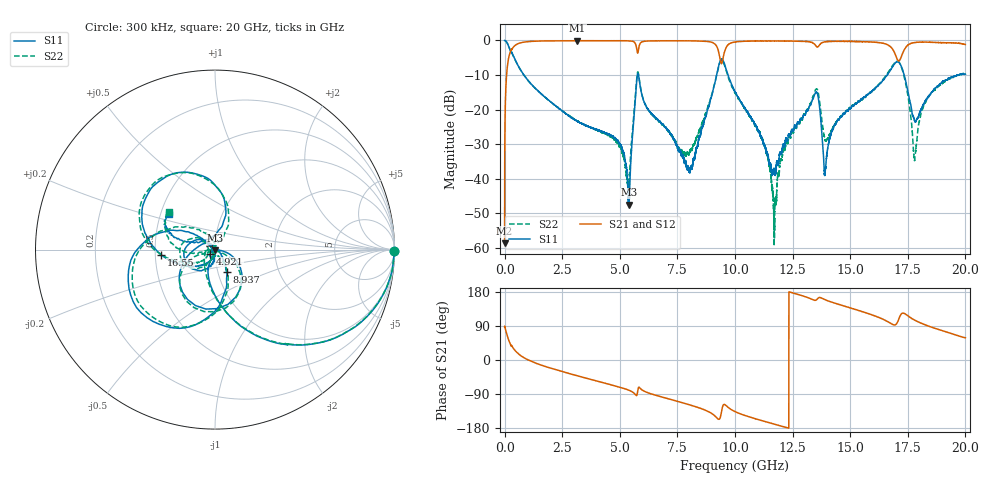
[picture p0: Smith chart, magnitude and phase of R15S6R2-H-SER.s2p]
!{R15S6R2}
!Johanson Technology Inc.
!www.johansontechnology.com
!Test Board Conditions:
!Substrate Type  RO4350B
!Substrate Thickness  20 mil
!Substrate Dk  3.66
!TL Type: GCPW
!TL Trace Width  34 mil
!TL Gap  10 mil
!Electrode orientation  Horizontal
!DUT TOPOLOGY	SERIES
!Mounting Pad LxW  26x52 mil
! Created Sat Feb  6 13:59:59 2021
# hz S ma R 50
! 2 Port Network Data from SP1.SP block
! freq  magS11  angS11  magS21  angS21  magS12  angS12  magS22  angS22
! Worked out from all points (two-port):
!   20001 points, 300 kHz to 20 GHz, reference 50 ohm
!   highest |S21| = -0.06 dB at 3.159 GHz (marker M1); lowest = -58.8 dB at 300 kHz (marker M2)
!   |S21| within 3 dB of the highest: 260.1 MHz to 5.749 GHz (5.489 GHz wide, 183 % of centre); 9.555 GHz to 16.89 GHz (7.333 GHz wide, 55.5 % of centre)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
!   lowest |S11| = -47.6 dB at 5.384 GHz (marker M3), VSWR 1.01, Z = 49.9 - j0.414 ohm
!   |S11| at or under -10 dB: 838.1 MHz to 5.761 GHz (4.923 GHz wide, 149 % of centre); 5.812 GHz to 9.202 GHz (3.39 GHz wide, 45.2 % of centre); 9.695 GHz to 16.61 GHz (6.913 GHz wide, 52.6 % of centre)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
!   |S22| runs from -59.6 to 0.0 dB; largest |S21 - S12| = 0.018
!   S11 on the Smith chart (normalised r, x): 300 kHz: open; 4.921 GHz: 0.95, -0.04; 8.937 GHz: 1.10, -0.28; 16.55 GHz: 0.54, -0.04; 20 GHz: 0.56, +0.25
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300000  1 -0.5  0.001149 87.1  0.001202 91.1  0.9991 -0.4
1.123e8  0.9157 -25.3  0.3965 64.5  0.3971 64.4  0.9157 -25.2
3.083e8  0.6718 -52.2  0.7351 37.7  0.7364 37.7  0.6722 -51.9
3.1593e9  0.06718 -112.5  0.9933 -41.7  0.992 -41.7  0.06796 -148.8
3.3343e9  0.06336 -112.8  0.992 -44.5  0.9911 -44.6  0.06383 -153.4
4.9213e9  0.03502 -140.2  0.9903 -70.5  0.9899 -70.5  0.033 -177.9
5.3843e9  0.004187 -97.7  0.9871 -79.5  0.9867 -79.5  0.008332 -69.1
5.7833e9  0.3347 -96.9  0.6607 -79.2  0.661 -79.2  0.3508 -98.4
6.6673e9  0.06965 150.8  0.9873 -94.9  0.9878 -94.8  0.0696 -159.8
8.0453e9  0.01305 38.6  0.986 -118.6  0.9862 -118.6  0.02498 -90.9
8.9373e9  0.14 -62.6  0.9521 -139.1  0.9521 -139.1  0.144 -62.0
9.4153e9  0.5422 -140.3  0.461 -136.4  0.4662 -136.2  0.5175 -139.5
1.00003e10  0.1805 146.6  0.9502 -136.2  0.9524 -136.2  0.173 136.0
1.17153e10  0.01276 -134.5  0.9824 -169.4  0.9839 -169.4  0.001761 -12.3
1.33343e10  0.1317 -120.1  0.9363 160.5  0.9392 160.4  0.1359 -131.0
1.39253e10  0.01381 -141.6  0.9562 158.7  0.9586 158.8  0.03526 175.3
1.65483e10  0.3001 -174.3  0.8899 103.7  0.8775 103.7  0.3093 -175.8
1.66673e10  0.3398 177.9  0.8513 99.8  0.8364 99.7  0.3535 177.9
1.72403e10  0.4049 97.0  0.6087 122.8  0.6006 122.9  0.3946 96.8
1.78083e10  0.06741 114.2  0.934 104.7  0.9377 105.0  0.01986 136.3
1.84053e10  0.1577 163.5  0.9438 89.3  0.9437 89.0  0.1522 -173.8
2e10  0.3234 141.7  0.8732 58.6  0.8651 58.2  0.33 140.1
